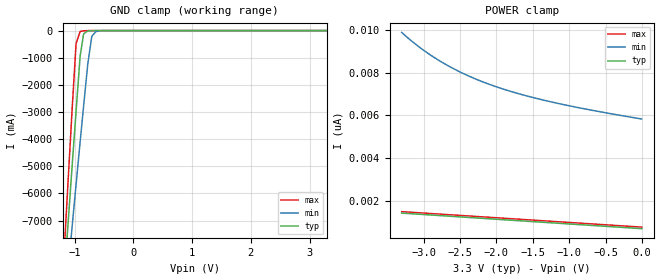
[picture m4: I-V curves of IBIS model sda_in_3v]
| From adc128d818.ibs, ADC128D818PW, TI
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[Model] sda_in_3v
Model_type Input
Vinh = 2.31V
Vinl = 0.99V
C_comp   1.61pF   0.89pF   1.90pF
[Voltage Range]   3.3V   3.0V   3.6V
[Temperature Range]   25.0   125.0   -40.0
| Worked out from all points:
|   GND clamp passes 1 mA (typ) near -0.65 V on its own axis
[GND Clamp]
-3.3V     -73.38A    -58.87A    -89.71A
-1.171V   -9.012A    -10.29A    -7.962A
-1.102V   -6.866A    -8.66A     -5.258A
-1.043V   -5.049A    -7.268A    -2.977A
-973.5mV  -2.968A    -5.666A    -472.9mA
-904.2mV  -931.6mA   -4.091A    -32.36mA
-844.8mV  -117.8mA   -2.767A    -7.285mA
-775.5mV  -16.37mA   -1.247A    -1.742mA
-706.2mV  -3.224mA   -212.7mA   -331.8uA
-636.9mV  -612.5uA   -37.79mA   -45.87uA
-438.9mV  -2.194uA   -495.7uA   -35.95nA
3.293V    722.4pA    0A         721.3pA
[POWER Clamp]
-3.3V     1.45nA     9.87nA     1.518nA
-3.161V   1.42nA     9.462nA    1.487nA
-3.033V   1.391nA    9.122nA    1.459nA
-2.765V   1.332nA    8.517nA    1.401nA
-2.627V   1.301nA    8.25nA     1.37nA
-2.458V   1.264nA    7.962nA    1.333nA
-2.3V     1.229nA    7.722nA    1.299nA
-2.092V   1.183nA    7.446nA    1.253nA
-1.696V   1.096nA    7.016nA    1.166nA
-1.261V   1nA        6.642nA    1.071nA
-696.3mV  876.6pA    6.248nA    947.5pA
-3.3mV    724.5pA    5.834nA    795.7pA
